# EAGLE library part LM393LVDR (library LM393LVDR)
Analog Comparators 1.65-V to 5.5-V, low voltage dual commodity comparator Source: Datasheet
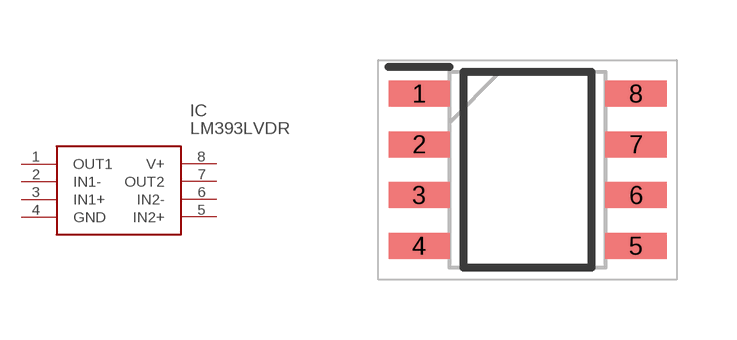
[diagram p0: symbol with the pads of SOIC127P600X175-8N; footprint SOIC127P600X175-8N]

Designator prefix IC

## LM393LVDR (Arrow_Part_Number: LM393LVDR; Arrow_Price-Stock: https://www.arrow.com/en/products/lm393lvdr/texas-instruments; Description: Analog Comparators 1.65-V to 5.5-V, low voltage dual commodity comparator; Height: 1.75mm; Manufacturer_Name: Texas Instruments; Manufacturer_Part_Number: LM393LVDR; Mouser_Part_Number: 595-LM393LVDR; Mouser_Price-Stock: https://www.mouser.co.uk/ProductDetail/Texas-Instruments/LM393LVDR?qs=zW32dvEIR3vk5%2FzEI25KTQ%3D%3D)  [SOIC127P600X175-8N]
1  OUT1
2  IN1-
3  IN1+
4  GND
5  IN2+
6  IN2-
7  OUT2
8  V+

## Footprint SOIC127P600X175-8N (pad centres in mm)
D(R-PDSO-G)
smd 1.528 x 0.65: 1 -2.711,1.905; 2 -2.711,0.635; 3 -2.711,-0.635; 4 -2.711,-1.905; 5 2.711,-1.905; 6 2.711,-0.635; 7 2.711,0.635; 8 2.711,1.905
